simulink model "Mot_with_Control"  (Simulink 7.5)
settings: Solver=ode3  StartTime=0.0  StopTime=inf  FixedStep=Ts  RelTol=1e-3
PreLoadFcn:
  | Ts=0.01;
libraries: simulink x6, arduino_lib x5

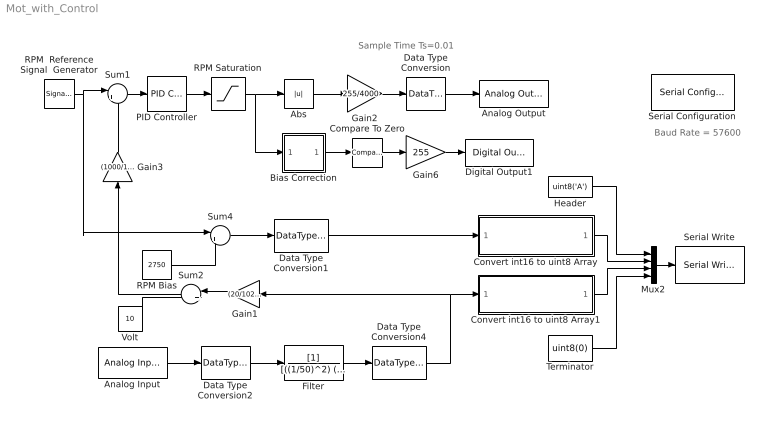
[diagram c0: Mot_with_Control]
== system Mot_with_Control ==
  note: Sample Time Ts=0.01
  note: Baud Rate = 57600
  Abs : Abs
  Analog Input : arduino_lib/Analog Input  SParameter1=0  SampleTime=Ts
  Analog Output : arduino_lib/Analog Output  SParameter1=6  SampleTime=-1
  Bias Correction : Subsystem
  Compare To Zero : simulink/Logic and Bit Operations/Compare To Zero  Priority=1  SystemSampleTime=-1  relop=>=  LogicOutDataTypeMode=uint8
  Convert int16 to uint8 Array : Subsystem
  Convert int16 to uint8 Array1 : Subsystem
  Data Type Conversion : DataTypeConversion  OutDataTypeMode=uint8  OutDataTypeStr=uint8
  Data Type Conversion1 : DataTypeConversion  OutDataTypeMode=int16  OutDataTypeStr=int16
  Data Type Conversion2 : DataTypeConversion  OutDataTypeMode=double  OutDataTypeStr=double
  Data Type Conversion4 : DataTypeConversion  OutDataTypeMode=int16  OutDataTypeStr=int16
  Digital Output1 : arduino_lib/Digital Output  SParameter1=13  SampleTime=-1
  Filter : TransferFcn  Denominator=[((1/50)^2) (2*0.707*(1/50)) 1]
  Gain1 : Gain  Gain=(20/1023)
  Gain2 : Gain  Gain=255/4000
  Gain3 : Gain  Gain=(1000/1.9)
  Gain6 : Gain  Gain=255
  Header : Constant  Value=uint8('A')
  Mux2 : Mux
  PID Controller : simulink/Continuous/PID Controller  DialogController=pidpack.PIDConfig.pidDDGCreate  DialogControllerArgs=DataTag0  SystemSampleTime=-1  Controller=PID  TimeDomain=Continuous-time  SampleTime=0.01  IntegratorMethod=Forward Euler  FilterMethod=Forward Euler  Form=Parallel  P=0.263336600419252  I=3.97797577428241  D=0  N=100  InitialConditionSource=internal  InitialConditionForIntegrator=0  InitialConditionForFilter=0  ExternalReset=none  LimitOutput=off  UpperSaturationLimit=inf  LowerSaturationLimit=-inf  LinearizeAsGain=off  AntiWindupMode=none  Kb=1  TrackingMode=off  Kt=1  PParamMin=[]  PParamMax=[]  IParamMin=[]  IParamMax=[]  DParamMin=[]  DParamMax=[]  NParamMin=[]  NParamMax=[]  KbParamMin=[]  KbParamMax=[]  KtParamMin=[]  KtParamMax=[]  POutMin=[]  POutMax=[]  IOutMin=[]  IOutMax=[]  DOutMin=[]  DOutMax=[]  NOutMin=[]  NOutMax=[]  KbOutMin=[]  KbOutMax=[]  KtOutMin=[]  KtOutMax=[]  IntegratorOutMin=[]  IntegratorOutMax=[]  FilterOutMin=[]  FilterOutMax=[]  SumOutMin=[]  SumOutMax=[]  SumI1OutMin=[]  SumI1OutMax=[]  SumI2OutMin=[]  SumI2OutMax=[]  SumI3OutMin=[]  SumI3OutMax=[]  SumDOutMin=[]  SumDOutMax=[]  SaturationOutMin=[]  SaturationOutMax=[]  IntegratorContinuousStateAttributes=''  IntegratorStateMustResolveToSignalObject=off  IntegratorRTWStateStorageClass=Auto  FilterContinuousStateAttributes=''  FilterStateMustResolveToSignalObject=off  FilterRTWStateStorageClass=Auto
  RPM  Reference Signal  Generator : SignalGenerator  WaveForm=square  Amplitude=2750  Frequency=1/10
  RPM Bias : Constant  Value=2750
  RPM Saturation : Saturate  UpperLimit=4000  LowerLimit=-4000
  Serial Configuration : arduino_lib/Serial Configuration  SParameter1=57600
  Serial Write : arduino_lib/Serial Write  SampleTime=-1
  Sum1 : Sum  Inputs=|+-
  Sum2 : Sum  Inputs=|+-
  Sum4 : Sum  Inputs=|++
  Terminator : Constant  Value=uint8(0)
  Volt : Constant  Value=10
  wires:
  Data Type Conversion/1 -> Analog Output/1
  Filter/1 -> Data Type Conversion4/1
  Data Type Conversion2/1 -> Filter/1
  Data Type Conversion4/1 -> Gain1/1, Convert int16 to uint8 Array1/1(From Analog In)
  Analog Input/1 -> Data Type Conversion2/1
  Gain1/1 -> Sum2/1
  Volt/1 -> Sum2/2
  Sum2/1 -> Gain3/1
  Gain2/1 -> Data Type Conversion/1
  RPM  Reference Signal  Generator/1 -> Sum1/1, Sum4/1
  Gain3/1 -> Sum1/2
  PID Controller/1 -> RPM Saturation/1
  Sum1/1 -> PID Controller/1
  RPM Saturation/1 -> Abs/1, Bias Correction/1(In)
  Abs/1 -> Gain2/1
  Header/1 -> Mux2/1
  Terminator/1 -> Mux2/4
  Mux2/1 -> Serial Write/1
  Sum4/1 -> Data Type Conversion1/1
  RPM Bias/1 -> Sum4/2
  Convert int16 to uint8 Array/1(To Serial) -> Mux2/2
  Convert int16 to uint8 Array1/1(To Serial) -> Mux2/3
  Data Type Conversion1/1 -> Convert int16 to uint8 Array/1(From Analog In)
  Compare To Zero/1 -> Gain6/1
  Gain6/1 -> Digital Output1/1
  Bias Correction/1(Out) -> Compare To Zero/1

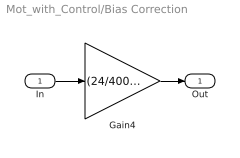
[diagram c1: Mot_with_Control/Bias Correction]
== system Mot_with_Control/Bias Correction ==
  In : Inport
  Gain4 : Gain  Gain=(24/4000)-12
  Out : Outport
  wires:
  Gain4/1 -> Out/1
  In/1 -> Gain4/1

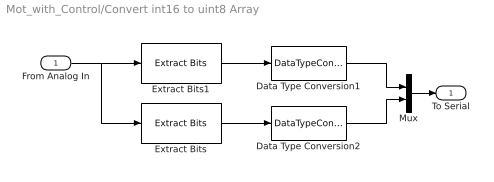
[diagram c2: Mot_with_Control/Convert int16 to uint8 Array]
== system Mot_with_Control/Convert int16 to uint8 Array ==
  From Analog In : Inport
  Data Type Conversion1 : DataTypeConversion  OutDataTypeMode=uint8  OutDataTypeStr=uint8  ConvertRealWorld=Stored Integer (SI)
  Data Type Conversion2 : DataTypeConversion  OutDataTypeMode=uint8  OutDataTypeStr=uint8  ConvertRealWorld=Stored Integer (SI)
  Extract Bits : simulink/Logic and Bit Operations/Extract Bits  SystemSampleTime=-1  bitsToExtract=Upper half  numBits=8  bitIdxRange=[0 7]  outScalingMode=Treat bit field as an integer
  Extract Bits1 : simulink/Logic and Bit Operations/Extract Bits  SystemSampleTime=-1  bitsToExtract=Lower half  numBits=8  bitIdxRange=[0 7]  outScalingMode=Treat bit field as an integer
  Mux : Mux  Inputs=2
  To Serial : Outport
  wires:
  Mux/1 -> To Serial/1
  Data Type Conversion2/1 -> Mux/2
  Data Type Conversion1/1 -> Mux/1
  Extract Bits/1 -> Data Type Conversion2/1
  Extract Bits1/1 -> Data Type Conversion1/1
  From Analog In/1 -> Extract Bits1/1, Extract Bits/1

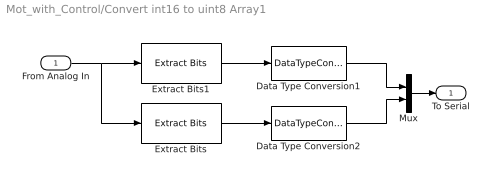
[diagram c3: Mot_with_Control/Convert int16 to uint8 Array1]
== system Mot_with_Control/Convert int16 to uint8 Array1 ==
  From Analog In : Inport
  Data Type Conversion1 : DataTypeConversion  OutDataTypeMode=uint8  OutDataTypeStr=uint8  ConvertRealWorld=Stored Integer (SI)
  Data Type Conversion2 : DataTypeConversion  OutDataTypeMode=uint8  OutDataTypeStr=uint8  ConvertRealWorld=Stored Integer (SI)
  Extract Bits : simulink/Logic and Bit Operations/Extract Bits  SystemSampleTime=-1  bitsToExtract=Upper half  numBits=8  bitIdxRange=[0 7]  outScalingMode=Treat bit field as an integer
  Extract Bits1 : simulink/Logic and Bit Operations/Extract Bits  SystemSampleTime=-1  bitsToExtract=Lower half  numBits=8  bitIdxRange=[0 7]  outScalingMode=Treat bit field as an integer
  Mux : Mux  Inputs=2
  To Serial : Outport
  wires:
  From Analog In/1 -> Extract Bits/1, Extract Bits1/1
  Extract Bits1/1 -> Data Type Conversion1/1
  Extract Bits/1 -> Data Type Conversion2/1
  Data Type Conversion1/1 -> Mux/1
  Data Type Conversion2/1 -> Mux/2
  Mux/1 -> To Serial/1
